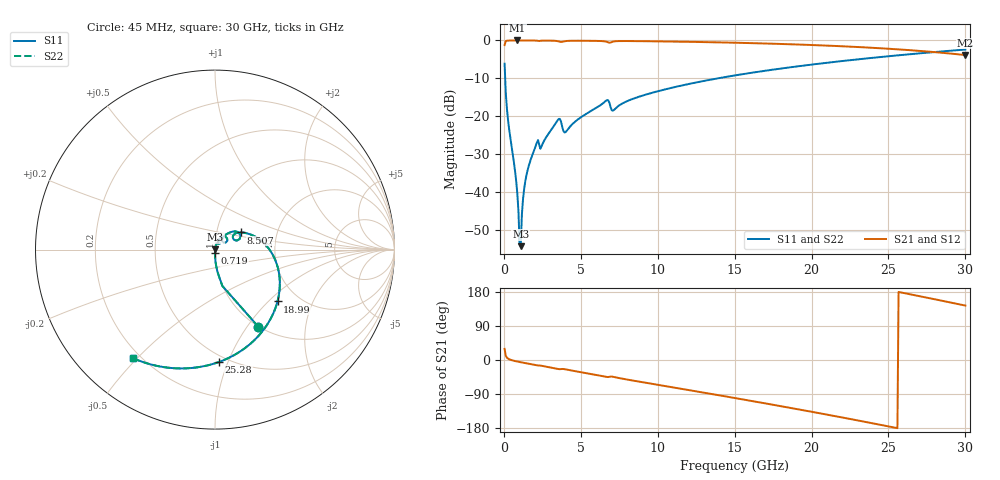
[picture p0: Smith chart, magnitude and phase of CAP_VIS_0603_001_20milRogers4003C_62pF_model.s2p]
! S-parameter model data by Modelithics Inc.  support@modelithics.com  813-866-6335  Tampa FL USA
! S-Parameter data specifications:
! Substrate: 20-mil Rogers 4003C, substrate thickness, H=0.508mm, Dielectric constant, Er=3.75
! PCB Mounting Pad Footprint: Pad width, PadW=0.90mm , Pad length, PadL=1.00mm , Pad gap, PadG (edge-to-edge)=1.00mm , Reference planes=3.0mm apart
! Created Wed Nov 18 13:29:48 2015
# hz S ma R 50
! 2 Port Network Data from SP1.SP block
! freq  magS11  angS11  magS21  angS21  magS12  angS12  magS22  angS22
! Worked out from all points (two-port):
!   401 points, 45 MHz to 30 GHz, reference 50 ohm
!   highest |S21| = -0.01 dB at 868.8 MHz (marker M1); lowest = -3.9 dB at 30 GHz (marker M2)
!   |S21| within 3 dB of the highest: start of sweep to 27.78 GHz
!   lowest |S11| = -54.3 dB at 1.093 GHz (marker M3), VSWR 1.00, Z = 50.1 + j0.155 ohm
!   |S11| at or under -10 dB: 83.15 MHz to 13.92 GHz (13.83 GHz wide, 198 % of centre)
!   |S22| runs from -54.3 to -2.4 dB; largest |S21 - S12| = 0
!   S11 on the Smith chart (normalised r, x): 45 MHz: 1.00, -1.13; 719 MHz: 1.00, -0.04; 8.507 GHz: 1.31, +0.26; 18.99 GHz: 1.57, -1.14; 25.28 GHz: 0.45, -0.93; 30 GHz: 0.17, -0.49
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4.5e7  0.4934 -60.7  0.8696 29.3  0.8696 29.3  0.4934 -60.7
2.696625e8  0.08837 -86.0  0.9956 3.6  0.9956 3.6  0.08837 -86.0
7.189875e8  0.01925 -90.3  0.999 -2.7  0.999 -2.7  0.01925 -90.3
8.687625e8  0.00969 -88.9  0.999 -4.1  0.999 -4.1  0.00969 -88.9
9.4365e8  0.005647 -85.4  0.999 -4.7  0.999 -4.7  0.005647 -85.4
1.093425e9  0.00193 53.3  0.9989 -5.9  0.9989 -5.9  0.00193 53.3
1.467862e9  0.01679 77.2  0.9985 -8.8  0.9985 -8.8  0.01679 77.2
2.066962e9  0.04048 71.9  0.9956 -13.3  0.9956 -13.3  0.04048 71.9
2.516288e9  0.0433 68.6  0.9946 -15.9  0.9946 -15.9  0.0433 68.6
3.489825e9  0.08841 55.3  0.9788 -23.5  0.9788 -23.5  0.08841 55.3
4.014038e9  0.06185 48.7  0.9803 -24.7  0.9803 -24.7  0.06185 48.7
5.062462e9  0.09862 54.9  0.9903 -32.6  0.9903 -32.6  0.09862 54.9
6.6351e9  0.1599 37.7  0.9647 -44.4  0.9647 -44.4  0.1599 37.7
7.159312e9  0.1211 35.0  0.971 -44.9  0.971 -44.9  0.1211 35.0
8.507288e9  0.1731 33.4  0.9797 -55.1  0.9797 -55.1  0.1731 33.4
1.007992e10  0.2156 23.0  0.9717 -66.0  0.9717 -66.0  0.2156 23.0
1.50225e10  0.3456 -11.1  0.9327 -100.4  0.9327 -100.4  0.3456 -11.1
1.899154e10  0.4524 -39.7  0.8851 -129.1  0.8851 -129.1  0.4524 -39.7
2.003996e10  0.4809 -47.4  0.8698 -136.9  0.8698 -136.9  0.4809 -47.4
2.505742e10  0.6202 -86.2  0.7756 -175.7  0.7756 -175.7  0.6202 -86.2
2.528209e10  0.6265 -88.0  0.7705 -177.5  0.7705 -177.5  0.6265 -88.0
3e10  0.7577 -126.9  0.6411 143.6  0.6411 143.6  0.7577 -126.9
